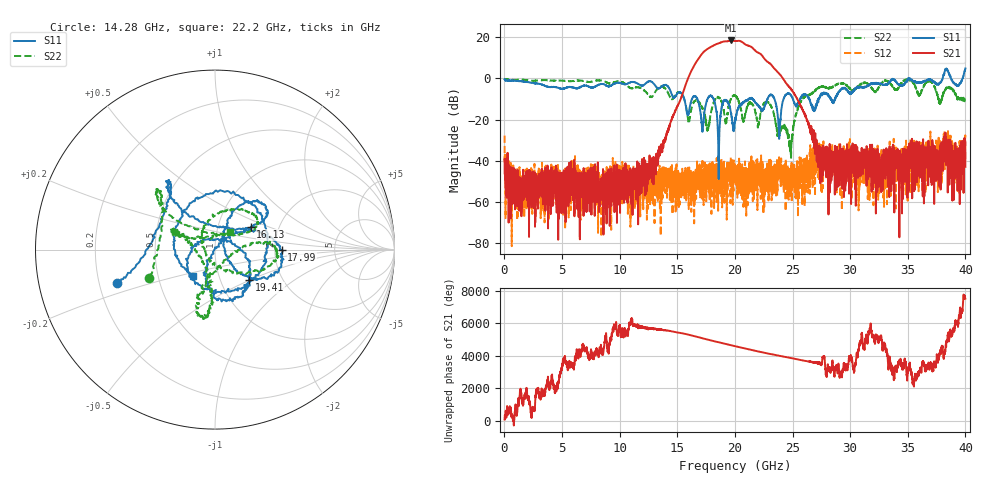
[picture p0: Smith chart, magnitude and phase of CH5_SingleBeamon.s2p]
!Keysight Technologies,N5245B,MY57181321,A.14.80.03
!Date: Thursday, March 28, 2024 17:40:52
!Correction: S11(C  2-Port  )
!S21(C  2-Port  )
!S12(C  2-Port  )
!S22(C  2-Port  )
!S2P File: Measurements: S11, S21, S12, S22:
# Hz S  RI  R 50
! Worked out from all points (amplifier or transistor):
!   4000 points, 10 MHz to 40 GHz, reference 50 ohm
!   highest |S21| = 18.4 dB at 19.67 GHz (marker M1)
!   |S21| within 3 dB of that: 17.96 GHz to 21.37 GHz (3.413 GHz wide, 17.4 % of centre)
!   unconditionally stable (mu >= 1): start of sweep to 35.05 GHz; 35.19 GHz to 38.03 GHz; 38.75 GHz to 39.75 GHz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
!   at 6.67 GHz: K = 4738.19, MAG = -37.2 dB, |S12| = -51.0 dB
!   at 20.01 GHz: K = 5.96, MAG = 18.9 dB, |S12| = -41.1 dB
!   at 40 GHz: K = -3340.82, MSG = -7.4 dB, |S12| = -28.1 dB
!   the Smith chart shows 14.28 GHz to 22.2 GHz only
!   S11 on the Smith chart (normalised r, x): 14.28 GHz: 0.27, -0.16; 16.13 GHz: 1.44, +0.38; 17.99 GHz: 2.18, -0.01; 19.41 GHz: 1.36, -0.49; 22.2 GHz: 0.75, -0.23
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1e7  0.9603 -0.0257  0.00352 0.0103  0.0296 -0.0284  -0.9799 0.0622
6.68e9  0.4192 0.4731  0.00166 0.00311  -0.00184 0.0026  0.8616 0.1769
1.334e10  -0.4027 -0.4093  -0.00875 -0.0119  0.001 -0.0014  -0.5445 -0.2142
1.428e10  -0.5472 -0.1886  -0.0468 0.051  0.00166 0.00152  -0.3658 -0.1568
1.613e10  0.1989 0.1257  -0.9032 -0.9849  0.000646 -0.00135  0.1108 0.08
1.696e10  0.0708 0.1682  0.7352 3.264  -0.00252 0.00218  0.1 0.2229
1.744e10  0.1593 -0.1394  4.663 -0.9158  -0.00394 -0.00163  -0.0713 0.0797
1.799e10  0.3714 -0.00135  -2.024 -5.535  -0.00436 -0.00745  0.1276 -0.133
1.844e10  0.091 0.0903  -6.788 0.887  0.000311 0.00367  0.3475 -0.0465
1.888e10  -0.0355 -0.2148  -1.107 7.522  -0.00188 -0.000765  0.2493 0.0412
1.941e10  0.1893 -0.1689  7.86 1.3  -0.000652 -0.00345  -0.0467 -0.1672
1.967e10  0.1357 0.00287  6.759 -4.776  -0.00222 -0.00255  -0.0936 -0.31
2.001e10  -0.0764 0.0455  -0.2785 -8.035  -0.00759 -0.00446  -0.063 -0.3864
2.05e10  -0.0363 -0.2155  -7.824 -1.119  0.00294 0.00529  -0.0216 -0.1813
2.102e10  0.2936 0.0106  -0.893 6.318  -0.000464 0.00144  -0.1731 0.0732
2.155e10  -0.0505 0.3097  5.14 1.606  -0.00104 0.000187  -0.2115 0.0841
2.22e10  -0.1208 -0.1481  0.4035 -3.913  -0.00148 0.00188  0.0861 0.097
2.27e10  0.2498 0.0475  -2.539 -0.9131  0.00126 0.00133  0.2111 0.1693
2.33e10  -0.0117 0.3682  -0.8697 1.69  0.00618 0.00126  0.1247 0.1049
2.667e10  0.2016 0.1111  0.0428 0.00343  0.0138 0.00287  0.3808 0.2035
3.334e10  0.6607 -0.3839  0.00315 7.11e-05  -0.000836 -0.0197  0.3162 -0.7511
4e10  0.2322 -1.724  0.00515 -0.00502  -0.00189 -0.0391  -0.0825 0.2545
